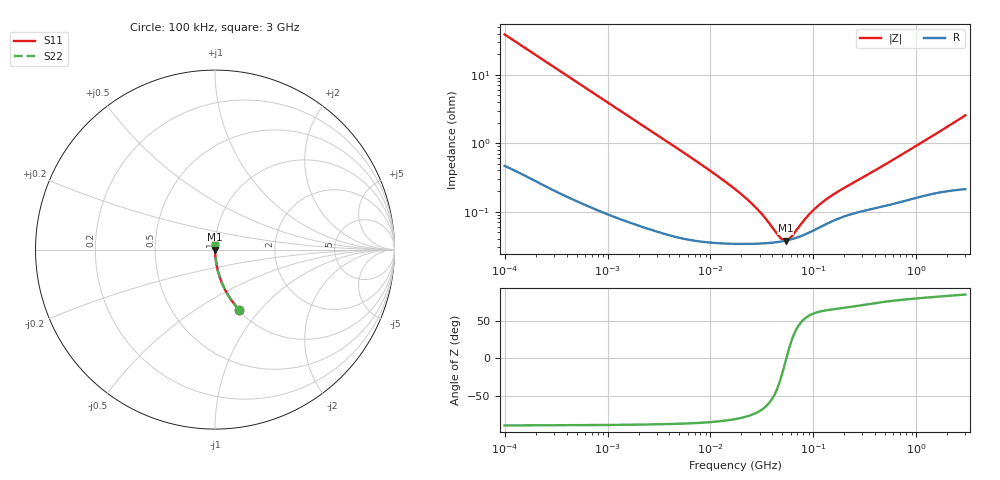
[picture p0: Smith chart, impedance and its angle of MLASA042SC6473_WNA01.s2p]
! MLASA042SC6473_WNA01  S-PARAMETER MODEL  ( Standard Model )
! Model Generated by TAIYO YUDEN Corporation (http://www.ty-top.com)
! Version 1.0
! TAIYO YUDEN Control No. 230906
! Copyright(c) 2023 TAIYO YUDEN CO.,LTD. All Rights Reserved.
! Product Description (link to TY-COMPAS)
! https://ds.yuden.co.jp/TYCOMPAS/or/detail?pn=MLASA042SC6473KWNA01&u=M
! Products Name : Multilayer Ceramic Capacitors
! Characteristics :
!  Capacitance : 0.047 [uF] , Rated Voltage : 4 [V] , TCC : X6S
!  Case Size : 0.4 x 0.2 / 0.016 x 0.008 [mm/inch] , Thickness : 0.2 / 0.008 [mm/inch]
!  (Conditions: Temperature = 25 [degC] , DC Bias Voltage = 0 [V])
! External Node Assignments :
!  1  o---| |---o  2
! GND o---------o GND
! Frequency Range : 100kHz  -  3GHz  [ 401 STEP ]
# MHZ S RI R 50
! Freq[MHz].  S11 Real  S11 Imag  S21 Real  S21 Imag  S12 Real  S12 Imag  S22 Real  S22 Imag
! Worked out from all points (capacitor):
!   401 points, 100 kHz to 3 GHz, reference 50 ohm
!   read as one part in series: C = 40.8 nF near 105.3 kHz
!   lowest |Z| = 37.7 mohm at 53.83 MHz (marker M1)
!   series resonance near 54.54 MHz, so ESL is about 210 pH
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0.1  0.1343 -0.3351  0.8657 0.3351  0.8657 0.3351  0.1343 -0.3351
0.1398  0.0751 -0.2571  0.9249 0.2571  0.9249 0.2571  0.0751 -0.2571
0.200542  0.0391 -0.1869  0.9609 0.1869  0.9609 0.1869  0.0391 -0.1869
0.327242  0.016 -0.1179  0.984 0.1179  0.984 0.1179  0.016 -0.1179
0.562235  0.0062 -0.0697  0.9938 0.0697  0.9938 0.0697  0.0062 -0.0697
1.18716  0.00194 -0.0334  0.9981 0.0334  0.9981 0.0334  0.00194 -0.0334
3.161081  0.000659 -0.0127  0.9993 0.0127  0.9993 0.0127  0.000659 -0.0127
9.331111  0.000373 -0.00422  0.9996 0.00422  0.9996 0.00422  0.000373 -0.00422
17.7727  0.000342 -0.00204  0.9997 0.00204  0.9997 0.00204  0.000342 -0.00204
23.59795  0.000339 -0.0014  0.9997 0.0014  0.9997 0.0014  0.000339 -0.0014
29.75839  0.000342 -0.000959  0.9997 0.000959  0.9997 0.000959  0.000342 -0.000959
47.32384  0.000363 -0.000212  0.9996 0.000212  0.9996 0.000212  0.000363 -0.000212
51.12795  0.000371 -9.6e-05  0.9996 9.6e-05  0.9996 9.6e-05  0.000371 -9.6e-05
53.83243  0.000376 -1.93e-05  0.9996 1.93e-05  0.9996 1.93e-05  0.000376 -1.93e-05
56.67997  0.000383 5.71e-05  0.9996 -5.71e-05  0.9996 -5.71e-05  0.000383 5.71e-05
61.23616  0.000394 0.000172  0.9996 -0.000172  0.9996 -0.000172  0.000394 0.000172
81.30716  0.000458 0.000594  0.9995 -0.000594  0.9995 -0.000594  0.000458 0.000594
97.38194  0.000519 0.000869  0.9995 -0.000869  0.9995 -0.000869  0.000519 0.000869
122.8043  0.000619 0.00123  0.9994 -0.00123  0.9994 -0.00123  0.000619 0.00123
158.9065  0.000745 0.00165  0.9993 -0.00165  0.9993 -0.00165  0.000745 0.00165
547.5153  0.00128 0.00516  0.9987 -0.00516  0.9987 -0.00516  0.00128 0.00516
3000  0.00277 0.0254  0.9972 -0.0254  0.9972 -0.0254  0.00277 0.0254
